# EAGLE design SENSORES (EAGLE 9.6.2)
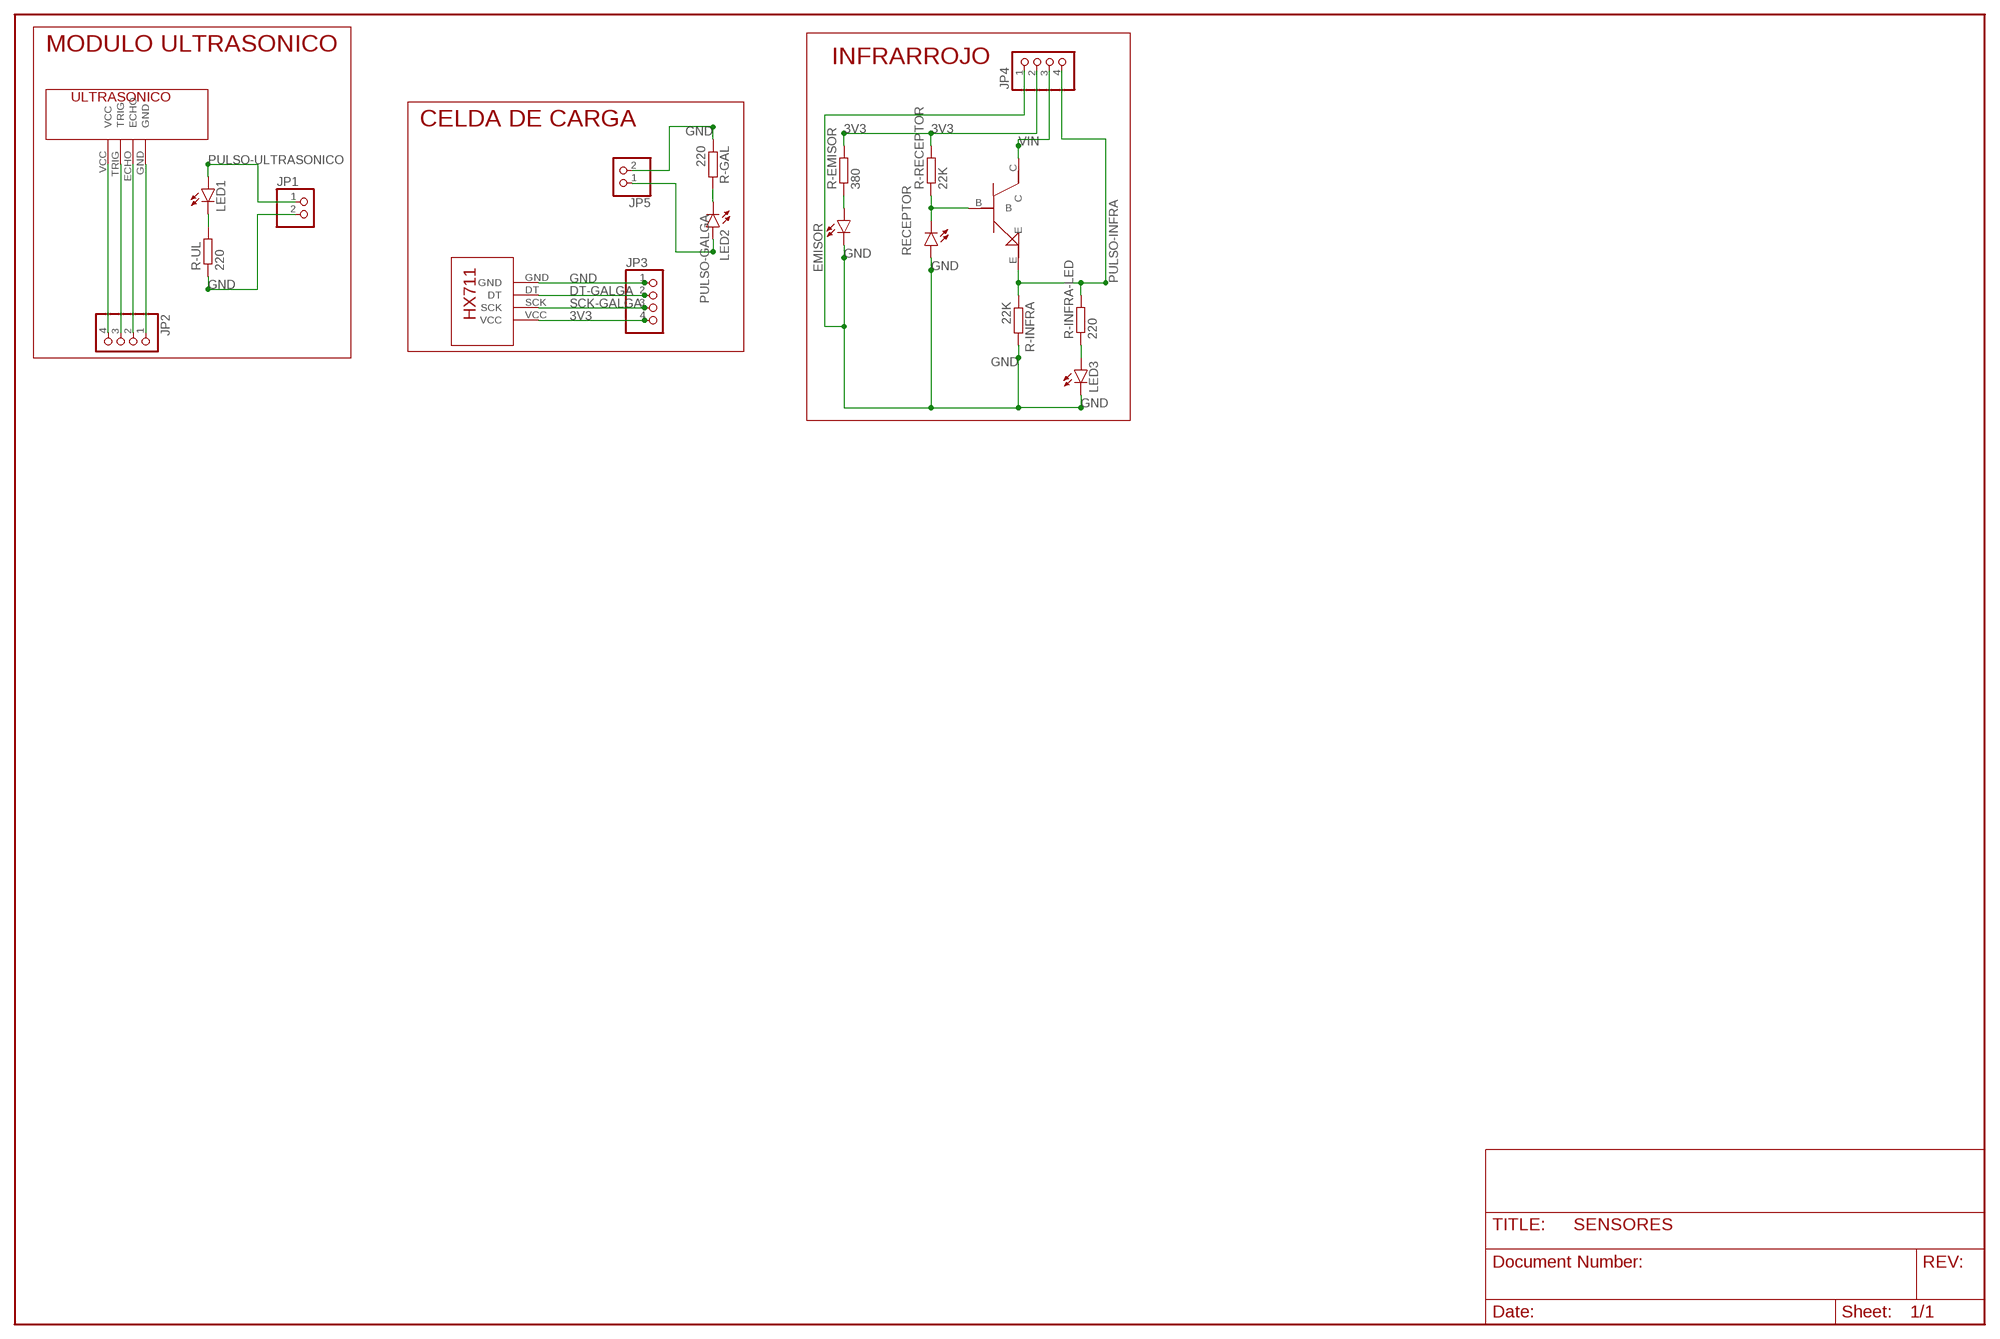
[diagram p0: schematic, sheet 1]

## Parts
EMISOR  LED3MM  [LED3MM]
JP1  PINHD-1X2  [1X02]
JP2  PINHD-1X4  [1X04]
JP3  PINHD-1X4  [1X04]
JP4  PINHD-1X4  [1X04]
JP5  PINHD-1X2  [1X02]
LED1  LED3MM  [LED3MM]
LED2  LED3MM  [LED3MM]
LED3  LED3MM  [LED3MM]
R-EMISOR  380  R-EU_0204/7  [0204/7]
R-GAL  220  R-EU_0204/7  [0204/7]
R-INFRA  22K  R-EU_0204/7  [0204/7]
R-INFRA-LED  220  R-EU_0204/7  [0204/7]
R-RECEPTOR  22K  R-EU_0204/7  [0204/7]
R-UL  220  R-EU_0204/7  [0204/7]
RECEPTOR  LED3MM  [LED3MM]
U$1  ULTRASONICO  [ULTRASONICO]
U$2  HX-711  [HX-711]
U$6  2N2222  [2N2222]

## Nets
3V3: JP3.4 JP4.2 R-EMISOR.2 R-RECEPTOR.2 U$2.VCC
DT-GALGA: JP3.2 U$2.DT
GND: EMISOR.K(C) JP1.2 JP3.1 JP4.1 JP5.2 LED3.K(C) R-GAL.1 R-INFRA.2 R-UL.1 RECEPTOR.A U$2.GND
N$1: LED1.K(C) R-UL.2
N$2: JP2.4 U$1.VCC
N$3: JP2.3 U$1.TRIG
N$4: JP2.2 U$1.ECHO
N$5: JP2.1 U$1.GND
N$8: LED2.K(C) R-GAL.2
N$20: EMISOR.A R-EMISOR.1
N$30: R-RECEPTOR.1 RECEPTOR.K(C) U$6.B
N$31: LED3.A R-INFRA-LED.1
PULSO-GALGA: JP5.1 LED2.A
PULSO-INFRA: JP4.4 R-INFRA-LED.2 R-INFRA.1 U$6.E
PULSO-ULTRASONICO: JP1.1 LED1.A
SCK-GALGA: JP3.3 U$2.SCK
VIN: JP4.3 U$6.C

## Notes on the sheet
- MODULO ULTRASONICO
- INFRARROJO
- CELDA DE CARGA

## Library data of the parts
EMISOR LED1-LED3 RECEPTOR = led:LED: LED
JP1 JP5 = pinhead:PINHD-1X2: PIN HEADER
JP2-JP4 = pinhead:PINHD-1X4: PIN HEADER
R-EMISOR R-GAL R-INFRA R-INFRA-LED R-RECEPTOR R-UL = rcl:R-EU_: RESISTOR, European symbol; SPICEPREFIX: R
U$1 = MODULAR:ULTRASONICO
U$2 = MODULAR:HX-711
U$6 = MODULAR:2N2222

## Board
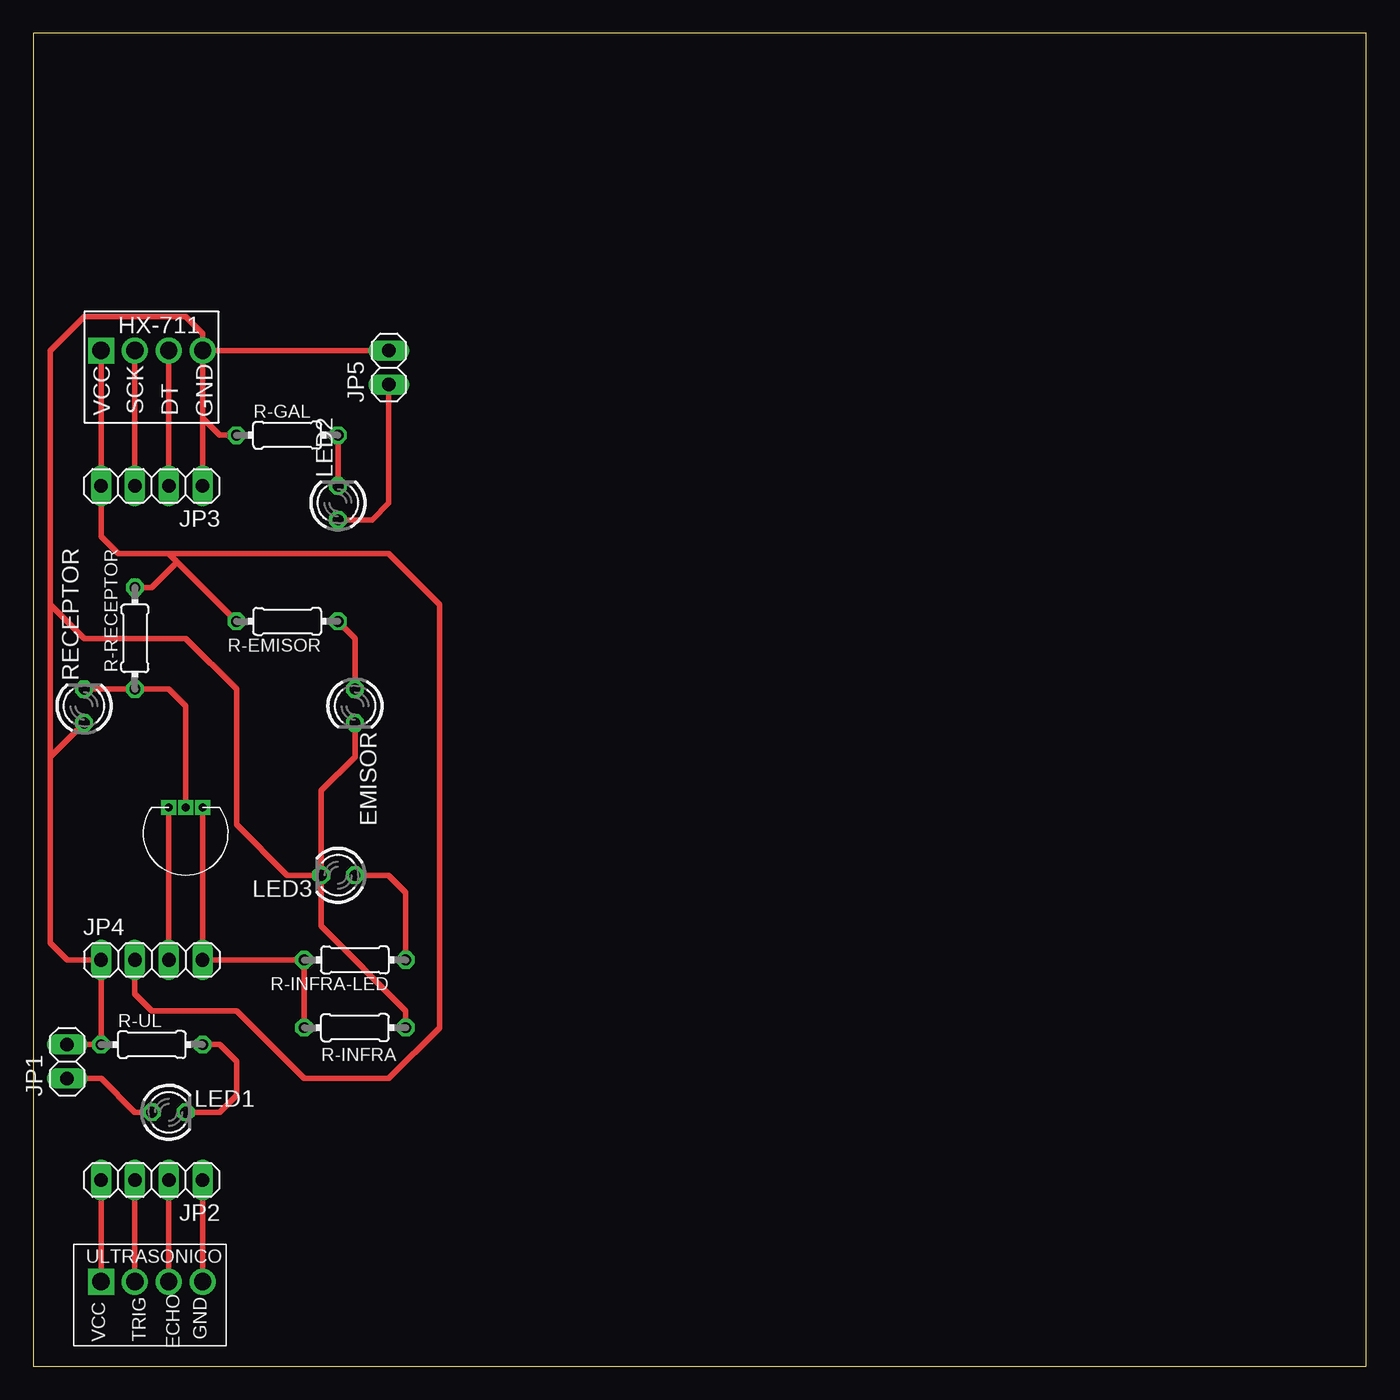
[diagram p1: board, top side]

Size 100 x 100 mm. Coordinates in mm from the lower left corner, seen from the top.
Outline: 0,0 100,0 100,100 0,100 0,0
Copper layers (1*16): Top 0.035mm / dielectric 1.5mm / Bottom 0.035mm
Design rules "default": minimum track width 6mil, minimum drill 0.35mm, track to track 6mil, track to pad 6mil, pad to pad 6mil, via to via 6mil, smd to smd 6mil, copper to edge 40mil, drill to drill 6mil, minimum pad ring 10mil, minimum via ring 8mil, stop-mask expansion 4mil, vias tented up to drill 0mil, thermal gap 10mil

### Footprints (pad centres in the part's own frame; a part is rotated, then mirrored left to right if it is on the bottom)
LED3MM = drill 0.813 octagon: A -1.27,0; K 1.27,0
1X02 = drill 1.016 long: 1 -1.27,0; 2 1.27,0
1X04 = drill 1.016 long: 1 -3.81,0; 2 -1.27,0; 3 1.27,0; 4 3.81,0
0204/7 = drill 0.813 octagon: 1 -3.81,0; 2 3.81,0
ULTRASONICO = drill 1.3: ECHO 2.54,0; GND 5.08,0; TRIG 0,0 | drill 1.3 square: VCC -2.54,0
HX-711 = drill 1.3: DT 2.54,0; GND 5.08,0; SCK 0,0 | drill 1.3 square: VCC -2.54,0
2N2222 = drill 0.6 square: B -2.54,1.27; C -2.54,0; E -2.54,2.54

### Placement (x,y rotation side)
EMISOR  24.13,49.53 270 top
JP1  2.54,22.86 90 top
JP2  8.89,13.97 180 top
JP3  8.89,66.04 180 top
JP4  8.89,30.48 0 top
JP5  26.67,74.93 90 top
LED1  10.16,19.05 0 top
LED2  22.86,64.77 90 top
LED3  22.86,36.83 180 top
R-EMISOR  19.05,55.88 180 top
R-GAL  19.05,69.85 0 top
R-INFRA  24.13,25.4 0 top
R-INFRA-LED  24.13,30.48 180 top
R-RECEPTOR  7.62,54.61 90 top
R-UL  8.89,24.13 0 top
RECEPTOR  3.81,49.53 90 top
U$1  7.62,6.35 0 top
U$2  7.62,76.2 0 top
U$6  10.16,39.37 270 top

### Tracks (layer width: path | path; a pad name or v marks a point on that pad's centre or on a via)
3V3
  Top 0.4: 10.16,60.96 6.35,60.96 5.08,62.23 JP3.4 U$2.VCC | JP4.2 7.62,27.94 8.89,26.67 15.24,26.67 20.32,21.59 26.67,21.59 30.48,25.4 30.48,57.15 26.67,60.96 10.16,60.96 | R-EMISOR.2 10.79,60.33 | 10.79,60.33 10.16,60.96 | R-RECEPTOR.2 8.89,58.42 10.79,60.33
DT-GALGA
  Top 0.4: U$2.DT JP3.2
GND
  Top 0.4: JP1.2 R-UL.1 JP4.1 2.54,30.48 1.27,31.75 1.27,45.72 | EMISOR.K 24.13,45.72 21.59,43.18 LED3.K | LED3.K 21.59,33.02 27.94,26.67 R-INFRA.2 | LED3.K 19.05,36.83 15.24,40.64 15.24,50.8 11.43,54.61 3.81,54.61 1.27,57.15 | U$2.GND 12.7,71.12 | 12.7,71.12 JP3.1 | JP5.2 U$2.GND | U$2.GND 12.7,77.47 11.43,78.74 3.81,78.74 1.27,76.2 1.27,57.15 | 1.27,45.72 1.27,57.15 | R-GAL.1 13.97,69.85 12.7,71.12 | RECEPTOR.A 1.27,45.72
N$1
  Top 0.4: R-UL.2 13.97,24.13 15.24,22.86 15.24,20.32 13.97,19.05 LED1.K
N$2
  Top 0.4: U$1.VCC JP2.4
N$3
  Top 0.4: U$1.TRIG JP2.3
N$4
  Top 0.4: U$1.ECHO JP2.2
N$5
  Top 0.4: U$1.GND JP2.1
N$8
  Top 0.4: LED2.K R-GAL.2
N$20
  Top 0.4: R-EMISOR.1 24.13,54.61 EMISOR.A
N$30
  Top 0.4: U$6.B 11.43,49.53 10.16,50.8 R-RECEPTOR.1 RECEPTOR.K
N$31
  Top 0.4: LED3.A 26.67,36.83 27.94,35.56 R-INFRA-LED.1
PULSO-GALGA
  Top 0.4: LED2.A 25.4,63.5 26.67,64.77 JP5.1
PULSO-INFRA
  Top 0.4: U$6.E JP4.4 R-INFRA-LED.2 R-INFRA.1
PULSO-ULTRASONICO
  Top 0.4: JP1.1 5.08,21.59 7.62,19.05 LED1.A
SCK-GALGA
  Top 0.4: U$2.SCK JP3.3
VIN
  Top 0.4: U$6.C JP4.3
